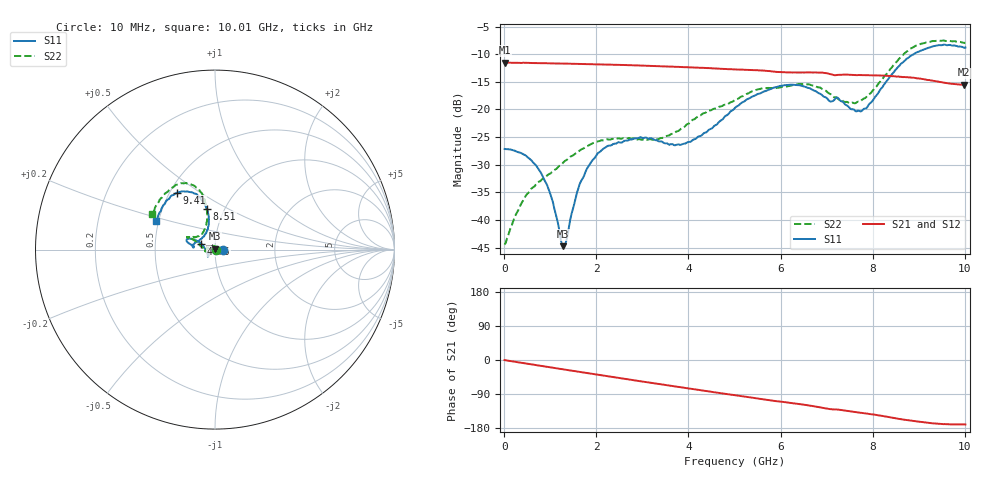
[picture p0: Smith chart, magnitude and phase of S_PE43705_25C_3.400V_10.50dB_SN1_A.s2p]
! Device ID: PE43705
! Serial: 1
! Insertion: A
! Impedance: 50 ohm
! Temp: 25C
! VDD: 3.400V
! Attenuation Step: 10.50dB
#  Hz  S  RI  R  50
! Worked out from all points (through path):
!   401 points, 10 MHz to 10.01 GHz, reference 50 ohm
!   highest |S21| = -11.50 dB at 10 MHz (marker M1); lowest = -15.5 dB at 9.985 GHz (marker M2)
!   group delay of S21, straight-line fit = 49 ps
!   lowest |S11| = -44.7 dB at 1.285 GHz (marker M3), VSWR 1.01, Z = 49.8 + j0.54 ohm
!   |S11| at or under -10 dB: start of sweep to 8.889 GHz
!   |S22| runs from -44.5 to -7.5 dB; largest |S21 - S12| = 0.0021
!   S11 on the Smith chart (normalised r, x): 10 MHz: 1.09, +0.00; 4.76 GHz: 0.86, +0.06; 8.51 GHz: 0.83, +0.40; 9.41 GHz: 0.55, +0.41; 10.01 GHz: 0.49, +0.18
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1e7  0.0439 5.23e-05  0.266 -0.00116  0.2663 -0.00114  0.00596 0.000348
4.1e8  0.0381 0.0104  0.2627 -0.036  0.2618 -0.0373  0.00304 0.0147
7.6e8  0.0242 0.0145  0.254 -0.067  0.254 -0.0669  -0.00773 0.0209
1.01e9  0.0119 0.0118  0.2464 -0.0878  0.2464 -0.0876  -0.0173 0.0199
1.285e9  -0.00201 0.00543  0.2365 -0.1087  0.2365 -0.1087  -0.0288 0.0163
1.685e9  -0.0213 -0.009  0.2183 -0.1378  0.2184 -0.1377  -0.0433 0.0063
2.21e9  -0.0354 -0.0287  0.1894 -0.171  0.1894 -0.1709  -0.0528 -0.00703
2.935e9  -0.0403 -0.0383  0.1414 -0.2064  0.1417 -0.2064  -0.0533 -0.00771
3.36e9  -0.0394 -0.0331  0.1105 -0.2203  0.1107 -0.2199  -0.054 -0.00412
3.985e9  -0.0502 -0.00609  0.0632 -0.2326  0.0634 -0.2323  -0.0726 0.0141
4.76e9  -0.0762 0.0333  0.00581 -0.2329  0.00631 -0.2328  -0.1008 0.0421
5.01e9  -0.0929 0.0455  -0.0117 -0.2301  -0.0115 -0.2303  -0.1118 0.049
5.985e9  -0.1515 0.0607  -0.0736 -0.2054  -0.0726 -0.2055  -0.1423 0.0692
6.685e9  -0.147 0.0355  -0.1127 -0.1844  -0.1125 -0.1846  -0.1497 0.0694
7.41e9  -0.1012 0.0436  -0.1429 -0.1494  -0.1423 -0.1498  -0.0867 0.0787
7.71e9  -0.0667 0.0704  -0.1543 -0.1349  -0.1537 -0.1352  -0.0652 0.0979
8.36e9  -0.0356 0.1918  -0.1759 -0.0978  -0.1753 -0.0986  -0.0462 0.2226
8.51e9  -0.0458 0.2276  -0.1786 -0.0862  -0.1779 -0.0876  -0.0547 0.2624
8.935e9  -0.1019 0.3094  -0.1828 -0.0604  -0.1822 -0.0591  -0.1198 0.3585
9.41e9  -0.2099 0.3173  -0.175 -0.0367  -0.1747 -0.0367  -0.2191 0.36
9.985e9  -0.32 0.1689  -0.1648 -0.0292  -0.165 -0.0291  -0.3432 0.2064
1.001e10  -0.3268 0.1599  -0.1652 -0.0291  -0.1662 -0.0295  -0.3505 0.1957
